(* Logix 5000 AddOnInstructionDefinition export Banner_Q90R2KU_Param_v4; software revision 33.00; part 3 of 3 *)
(* tags used below, declared in another part *)
   Q90RKU : Banner_Q90R2KU_v4;
   Port_Data : Banner_IOL_Port_v4;
   Port : DINT;
   Local_Control : DINT;
   Command_Being_Processed : BOOL;
   Update_Archive : BOOL;
   Index_Write_Inprocess : DINT;
   Inprocess_Index : DINT;
(* Banner_Q90R2KU_Param_v4, continued *)

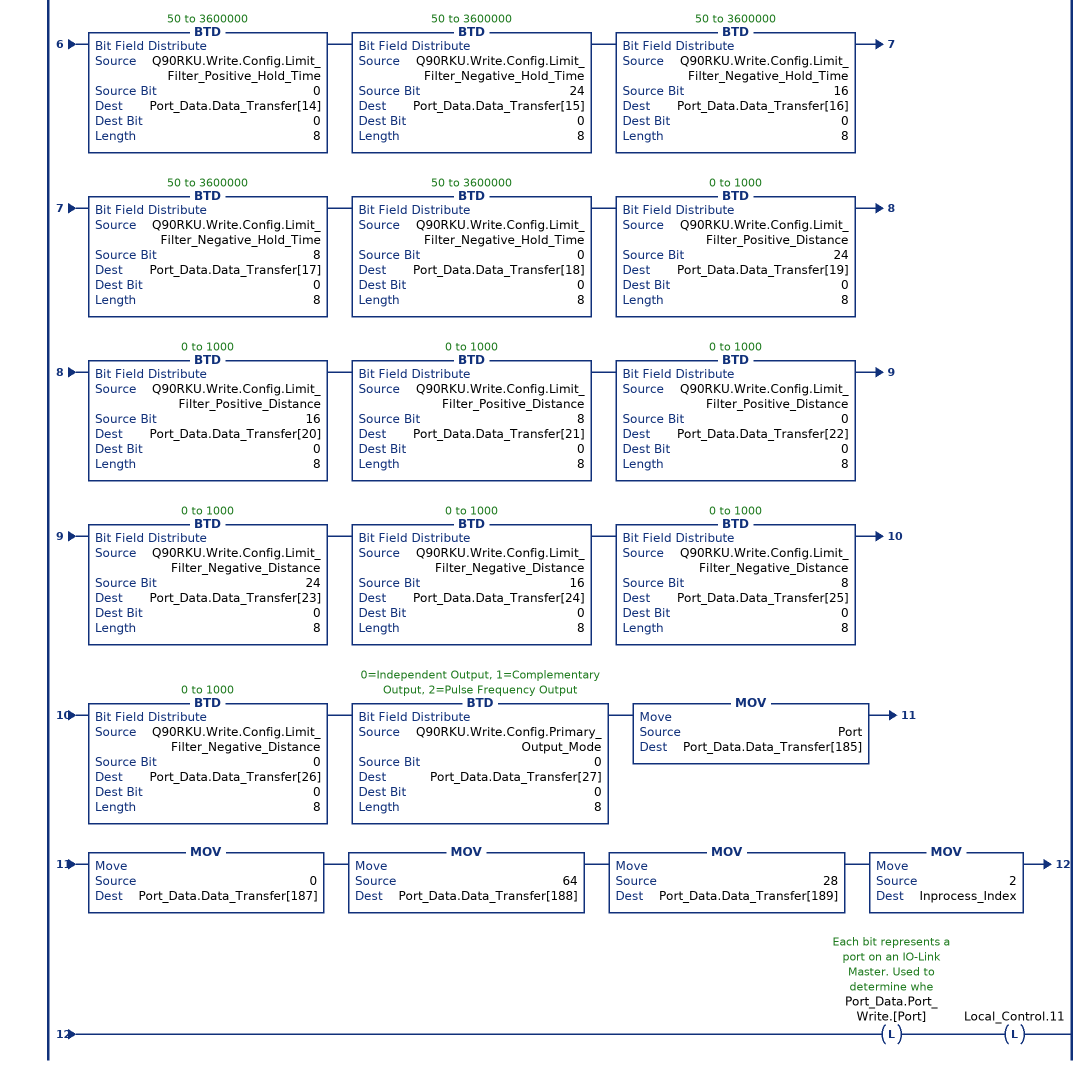
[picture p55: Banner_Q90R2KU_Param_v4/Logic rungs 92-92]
   // ************************************************************************************************************
   // Section of AOI that controls writing of the Configuration parameter (index 64).
   // ************************************************************************************************************
   92: XIC(Q90RKU.Initial_Global_Read)XIO(Command_Being_Processed)XIO(Local_Control.11)EQU(Q90RKU.Command,44)OTL(Command_Being_Processed)MOV(0,Port_Data.Data_Transfer[0])MOV(0,Port_Data.Data_Transfer[1])BTD(Q90RKU.Write.Config.Response_Speed,0,Port_Data.Data_Transfer[0],0,8)BTD(Q90RKU.Write.Config.Detection_Sensitivity,0,Port_Data.Data_Transfer[1],0,8)BTD(Q90RKU.Write.Config.LEDs_Disabled,0,Port_Data.Data_Transfer[2],0,8)BTD(Q90RKU.Write.Config.Output_Polarity,0,Port_Data.Data_Transfer[3],0,8)BTD(Q90RKU.Write.Config.PD_Measurement,0,Port_Data.Data_Transfer[4],0,8)BTD(Q90RKU.Write.Config.Remote_Input_Mode,0,Port_Data.Data_Transfer[5],0,8)BTD(Q90RKU.Write.Config.Amplitude_Threshold,24,Port_Data.Data_Transfer[6],0,8)BTD(Q90RKU.Write.Config.Amplitude_Threshold,16,Port_Data.Data_Transfer[7],0,8)BTD(Q90RKU.Write.Config.Amplitude_Threshold,8,Port_Data.Data_Transfer[8],0,8)BTD(Q90RKU.Write.Config.Amplitude_Threshold,0,Port_Data.Data_Transfer[9],0,8)BTD(Q90RKU.Write.Config.Limit_Filter_Enabled,0,Port_Data.Data_Transfer[10],0,8)BTD(Q90RKU.Write.Config.Limit_Filter_Positive_Hold_Time,24,Port_Data.Data_Transfer[11],0,8)BTD(Q90RKU.Write.Config.Limit_Filter_Positive_Hold_Time,16,Port_Data.Data_Transfer[12],0,8)BTD(Q90RKU.Write.Config.Limit_Filter_Positive_Hold_Time,8,Port_Data.Data_Transfer[13],0,8)BTD(Q90RKU.Write.Config.Limit_Filter_Positive_Hold_Time,0,Port_Data.Data_Transfer[14],0,8)BTD(Q90RKU.Write.Config.Limit_Filter_Negative_Hold_Time,24,Port_Data.Data_Transfer[15],0,8)BTD(Q90RKU.Write.Config.Limit_Filter_Negative_Hold_Time,16,Port_Data.Data_Transfer[16],0,8)BTD(Q90RKU.Write.Config.Limit_Filter_Negative_Hold_Time,8,Port_Data.Data_Transfer[17],0,8)BTD(Q90RKU.Write.Config.Limit_Filter_Negative_Hold_Time,0,Port_Data.Data_Transfer[18],0,8)BTD(Q90RKU.Write.Config.Limit_Filter_Positive_Distance,24,Port_Data.Data_Transfer[19],0,8)BTD(Q90RKU.Write.Config.Limit_Filter_Positive_Distance,16,Port_Data.Data_Transfer[20],0,8)BTD(Q90RKU.Write.Config.Limit_Filter_Positive_Distance,8,Port_Data.Data_Transfer[21],0,8)BTD(Q90RKU.Write.Config.Limit_Filter_Positive_Distance,0,Port_Data.Data_Transfer[22],0,8)BTD(Q90RKU.Write.Config.Limit_Filter_Negative_Distance,24,Port_Data.Data_Transfer[23],0,8)BTD(Q90RKU.Write.Config.Limit_Filter_Negative_Distance,16,Port_Data.Data_Transfer[24],0,8)BTD(Q90RKU.Write.Config.Limit_Filter_Negative_Distance,8,Port_Data.Data_Transfer[25],0,8)BTD(Q90RKU.Write.Config.Limit_Filter_Negative_Distance,0,Port_Data.Data_Transfer[26],0,8)BTD(Q90RKU.Write.Config.Primary_Output_Mode,0,Port_Data.Data_Transfer[27],0,8)MOV(Port,Port_Data.Data_Transfer[185])MOV(0,Port_Data.Data_Transfer[187])MOV(64,Port_Data.Data_Transfer[188])MOV(28,Port_Data.Data_Transfer[189])MOV(2,Inprocess_Index)OTL(Port_Data.Port_Write.[Port])OTL(Local_Control.11);
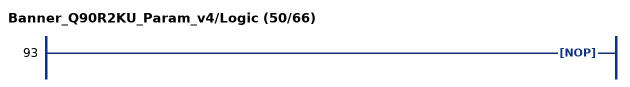
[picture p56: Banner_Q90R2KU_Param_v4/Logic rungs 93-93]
   93: NOP();
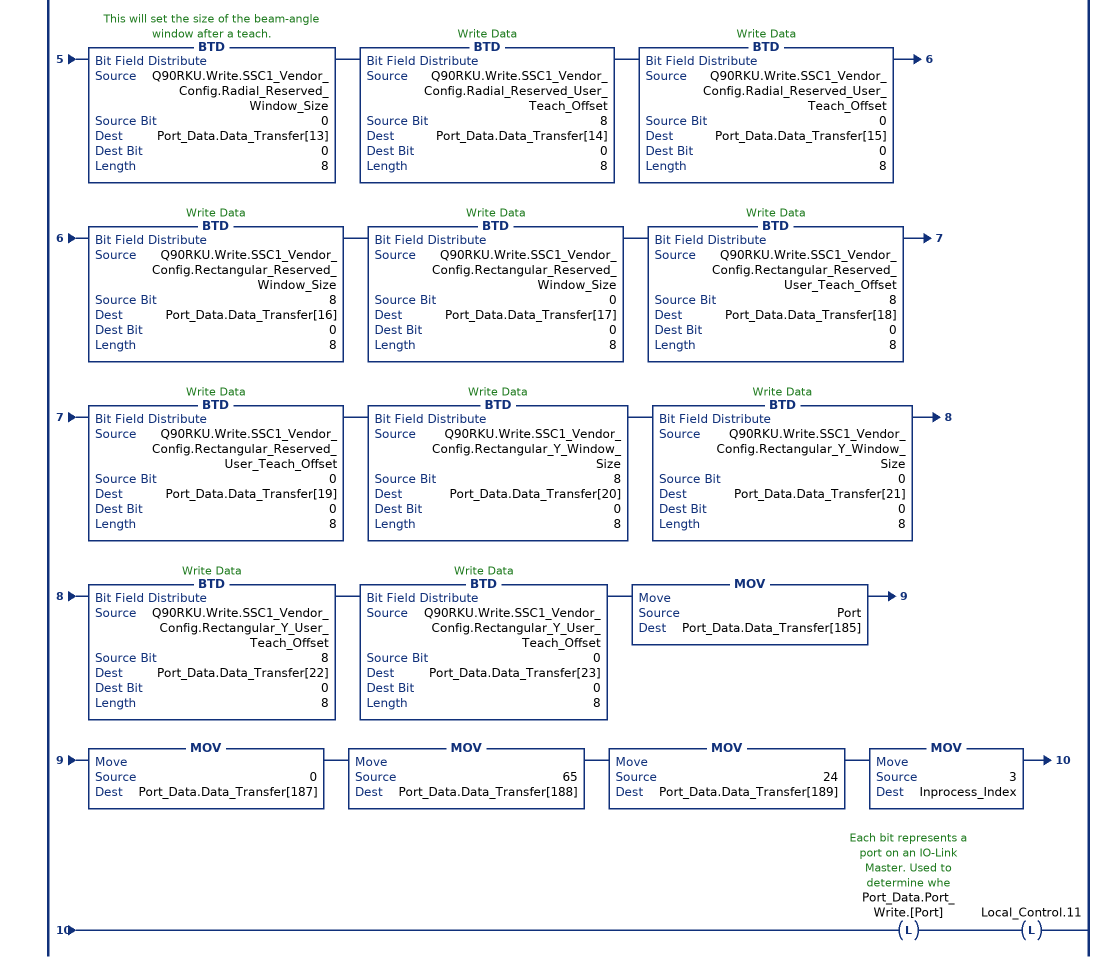
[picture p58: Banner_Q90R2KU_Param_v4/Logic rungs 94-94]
   // ************************************************************************************************************
   // Section of AOI that controls writing of the SSC1 Vendor Specific Configuration parameter (index 65).
   // ************************************************************************************************************
   94: XIC(Q90RKU.Initial_Global_Read)XIO(Command_Being_Processed)XIO(Local_Control.11)EQU(Q90RKU.Command,45)OTL(Command_Being_Processed)BTD(Q90RKU.Write.SSC1_Vendor_Config.Delay_On,24,Port_Data.Data_Transfer[0],0,8)BTD(Q90RKU.Write.SSC1_Vendor_Config.Delay_On,16,Port_Data.Data_Transfer[1],0,8)BTD(Q90RKU.Write.SSC1_Vendor_Config.Delay_On,8,Port_Data.Data_Transfer[2],0,8)BTD(Q90RKU.Write.SSC1_Vendor_Config.Delay_On,0,Port_Data.Data_Transfer[3],0,8)BTD(Q90RKU.Write.SSC1_Vendor_Config.Delay_Off,24,Port_Data.Data_Transfer[4],0,8)BTD(Q90RKU.Write.SSC1_Vendor_Config.Delay_Off,16,Port_Data.Data_Transfer[5],0,8)BTD(Q90RKU.Write.SSC1_Vendor_Config.Delay_Off,8,Port_Data.Data_Transfer[6],0,8)BTD(Q90RKU.Write.SSC1_Vendor_Config.Delay_Off,0,Port_Data.Data_Transfer[7],0,8)BTD(Q90RKU.Write.SSC1_Vendor_Config.Radial_Distance_Window_Size,8,Port_Data.Data_Transfer[8],0,8)BTD(Q90RKU.Write.SSC1_Vendor_Config.Radial_Distance_Window_Size,0,Port_Data.Data_Transfer[9],0,8)BTD(Q90RKU.Write.SSC1_Vendor_Config.Radial_Distance_User_Teach_Offset,8,Port_Data.Data_Transfer[10],0,8)BTD(Q90RKU.Write.SSC1_Vendor_Config.Radial_Distance_User_Teach_Offset,0,Port_Data.Data_Transfer[11],0,8)BTD(Q90RKU.Write.SSC1_Vendor_Config.Radial_Reserved_Window_Size,8,Port_Data.Data_Transfer[12],0,8)BTD(Q90RKU.Write.SSC1_Vendor_Config.Radial_Reserved_Window_Size,0,Port_Data.Data_Transfer[13],0,8)BTD(Q90RKU.Write.SSC1_Vendor_Config.Radial_Reserved_User_Teach_Offset,8,Port_Data.Data_Transfer[14],0,8)BTD(Q90RKU.Write.SSC1_Vendor_Config.Radial_Reserved_User_Teach_Offset,0,Port_Data.Data_Transfer[15],0,8)BTD(Q90RKU.Write.SSC1_Vendor_Config.Rectangular_Reserved_Window_Size,8,Port_Data.Data_Transfer[16],0,8)BTD(Q90RKU.Write.SSC1_Vendor_Config.Rectangular_Reserved_Window_Size,0,Port_Data.Data_Transfer[17],0,8)BTD(Q90RKU.Write.SSC1_Vendor_Config.Rectangular_Reserved_User_Teach_Offset,8,Port_Data.Data_Transfer[18],0,8)BTD(Q90RKU.Write.SSC1_Vendor_Config.Rectangular_Reserved_User_Teach_Offset,0,Port_Data.Data_Transfer[19],0,8)BTD(Q90RKU.Write.SSC1_Vendor_Config.Rectangular_Y_Window_Size,8,Port_Data.Data_Transfer[20],0,8)BTD(Q90RKU.Write.SSC1_Vendor_Config.Rectangular_Y_Window_Size,0,Port_Data.Data_Transfer[21],0,8)BTD(Q90RKU.Write.SSC1_Vendor_Config.Rectangular_Y_User_Teach_Offset,8,Port_Data.Data_Transfer[22],0,8)BTD(Q90RKU.Write.SSC1_Vendor_Config.Rectangular_Y_User_Teach_Offset,0,Port_Data.Data_Transfer[23],0,8)MOV(Port,Port_Data.Data_Transfer[185])MOV(0,Port_Data.Data_Transfer[187])MOV(65,Port_Data.Data_Transfer[188])MOV(24,Port_Data.Data_Transfer[189])MOV(3,Inprocess_Index)OTL(Port_Data.Port_Write.[Port])OTL(Local_Control.11);
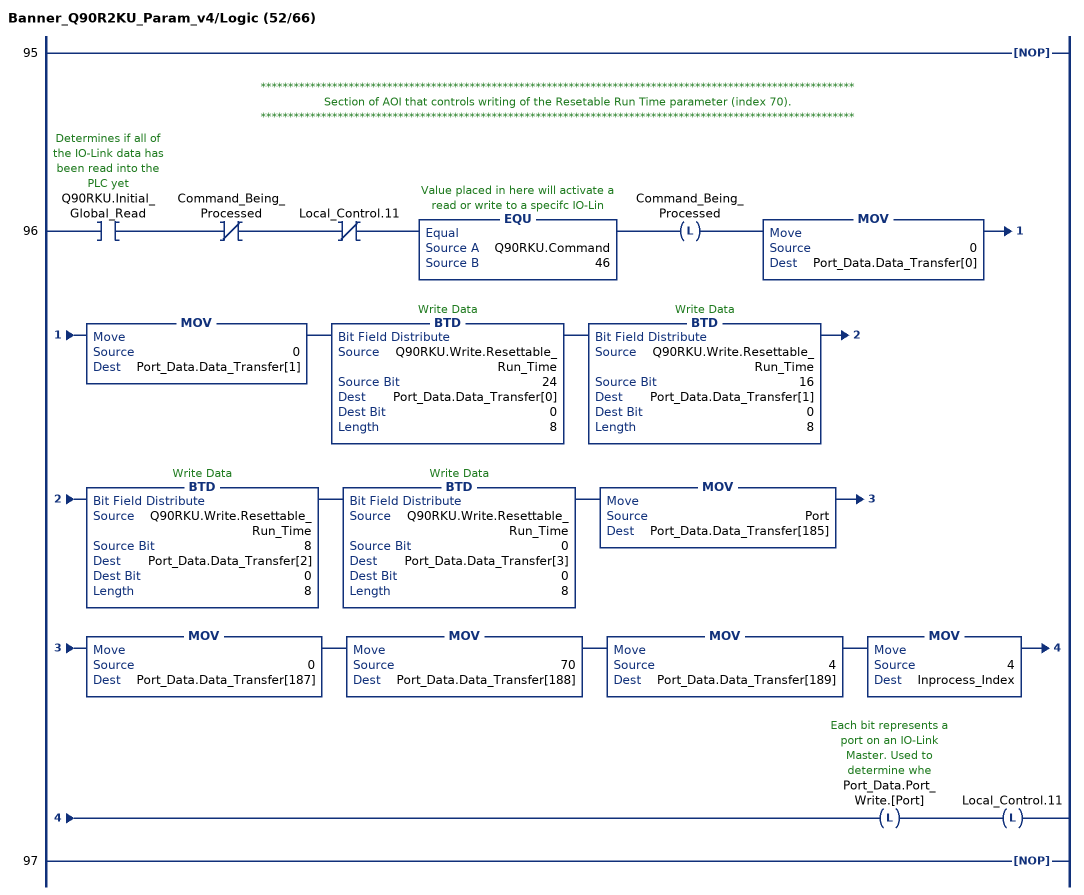
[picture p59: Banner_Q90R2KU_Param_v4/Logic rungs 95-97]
   95: NOP();
   // ************************************************************************************************************
   // Section of AOI that controls writing of the Resetable Run Time parameter (index 70).
   // ************************************************************************************************************
   96: XIC(Q90RKU.Initial_Global_Read)XIO(Command_Being_Processed)XIO(Local_Control.11)EQU(Q90RKU.Command,46)OTL(Command_Being_Processed)MOV(0,Port_Data.Data_Transfer[0])MOV(0,Port_Data.Data_Transfer[1])BTD(Q90RKU.Write.Resettable_Run_Time,24,Port_Data.Data_Transfer[0],0,8)BTD(Q90RKU.Write.Resettable_Run_Time,16,Port_Data.Data_Transfer[1],0,8)BTD(Q90RKU.Write.Resettable_Run_Time,8,Port_Data.Data_Transfer[2],0,8)BTD(Q90RKU.Write.Resettable_Run_Time,0,Port_Data.Data_Transfer[3],0,8)MOV(Port,Port_Data.Data_Transfer[185])MOV(0,Port_Data.Data_Transfer[187])MOV(70,Port_Data.Data_Transfer[188])MOV(4,Port_Data.Data_Transfer[189])MOV(4,Inprocess_Index)OTL(Port_Data.Port_Write.[Port])OTL(Local_Control.11);
   97: NOP();
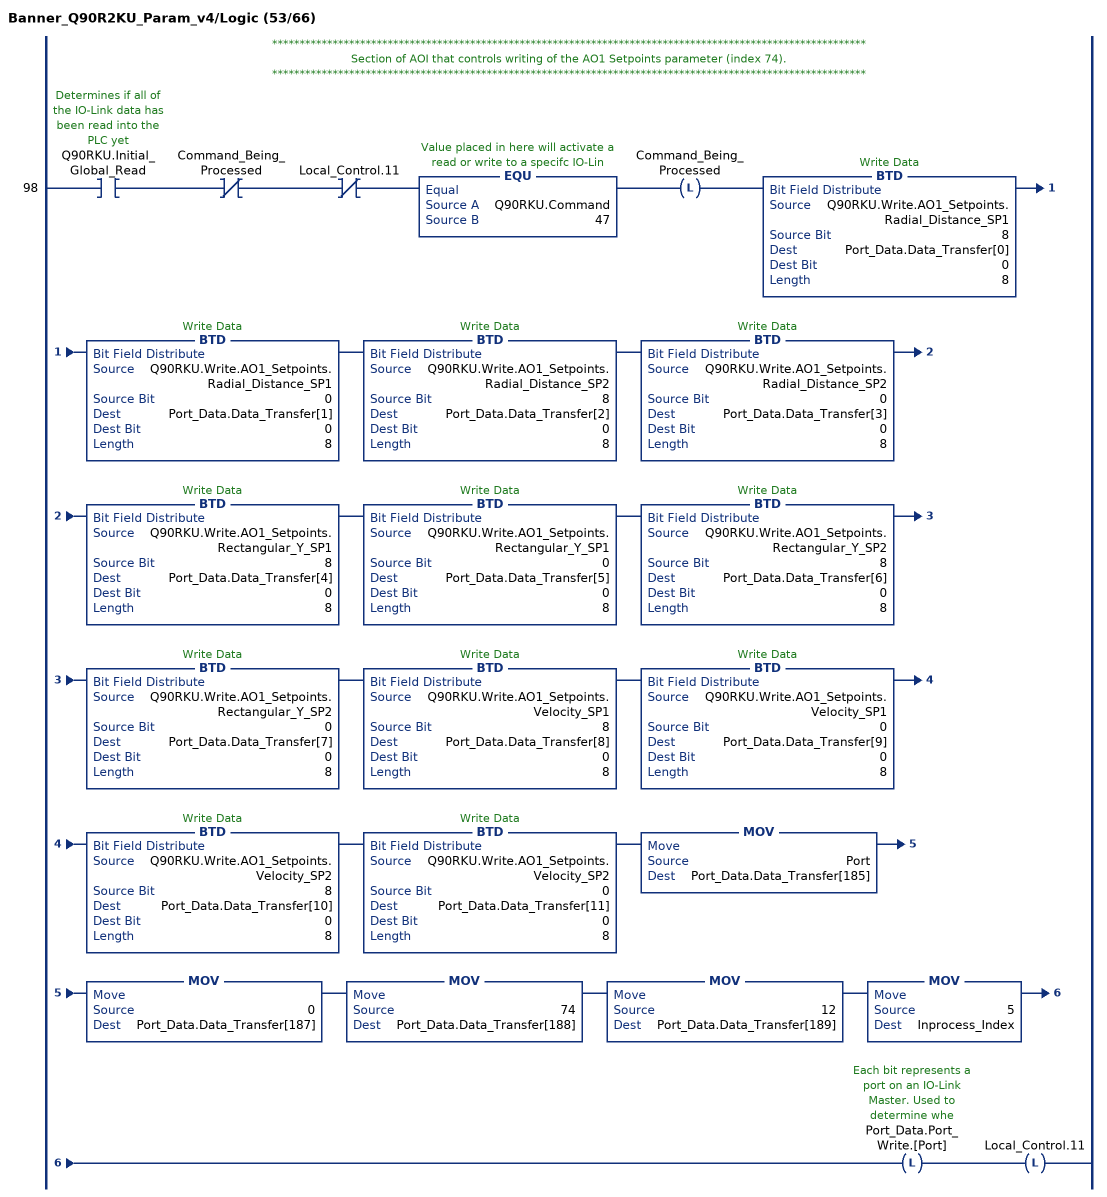
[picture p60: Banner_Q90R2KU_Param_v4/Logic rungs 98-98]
   // ************************************************************************************************************
   // Section of AOI that controls writing of the AO1 Setpoints parameter (index 74).
   // ************************************************************************************************************
   98: XIC(Q90RKU.Initial_Global_Read)XIO(Command_Being_Processed)XIO(Local_Control.11)EQU(Q90RKU.Command,47)OTL(Command_Being_Processed)BTD(Q90RKU.Write.AO1_Setpoints.Radial_Distance_SP1,8,Port_Data.Data_Transfer[0],0,8)BTD(Q90RKU.Write.AO1_Setpoints.Radial_Distance_SP1,0,Port_Data.Data_Transfer[1],0,8)BTD(Q90RKU.Write.AO1_Setpoints.Radial_Distance_SP2,8,Port_Data.Data_Transfer[2],0,8)BTD(Q90RKU.Write.AO1_Setpoints.Radial_Distance_SP2,0,Port_Data.Data_Transfer[3],0,8)BTD(Q90RKU.Write.AO1_Setpoints.Rectangular_Y_SP1,8,Port_Data.Data_Transfer[4],0,8)BTD(Q90RKU.Write.AO1_Setpoints.Rectangular_Y_SP1,0,Port_Data.Data_Transfer[5],0,8)BTD(Q90RKU.Write.AO1_Setpoints.Rectangular_Y_SP2,8,Port_Data.Data_Transfer[6],0,8)BTD(Q90RKU.Write.AO1_Setpoints.Rectangular_Y_SP2,0,Port_Data.Data_Transfer[7],0,8)BTD(Q90RKU.Write.AO1_Setpoints.Velocity_SP1,8,Port_Data.Data_Transfer[8],0,8)BTD(Q90RKU.Write.AO1_Setpoints.Velocity_SP1,0,Port_Data.Data_Transfer[9],0,8)BTD(Q90RKU.Write.AO1_Setpoints.Velocity_SP2,8,Port_Data.Data_Transfer[10],0,8)BTD(Q90RKU.Write.AO1_Setpoints.Velocity_SP2,0,Port_Data.Data_Transfer[11],0,8)MOV(Port,Port_Data.Data_Transfer[185])MOV(0,Port_Data.Data_Transfer[187])MOV(74,Port_Data.Data_Transfer[188])MOV(12,Port_Data.Data_Transfer[189])MOV(5,Inprocess_Index)OTL(Port_Data.Port_Write.[Port])OTL(Local_Control.11);
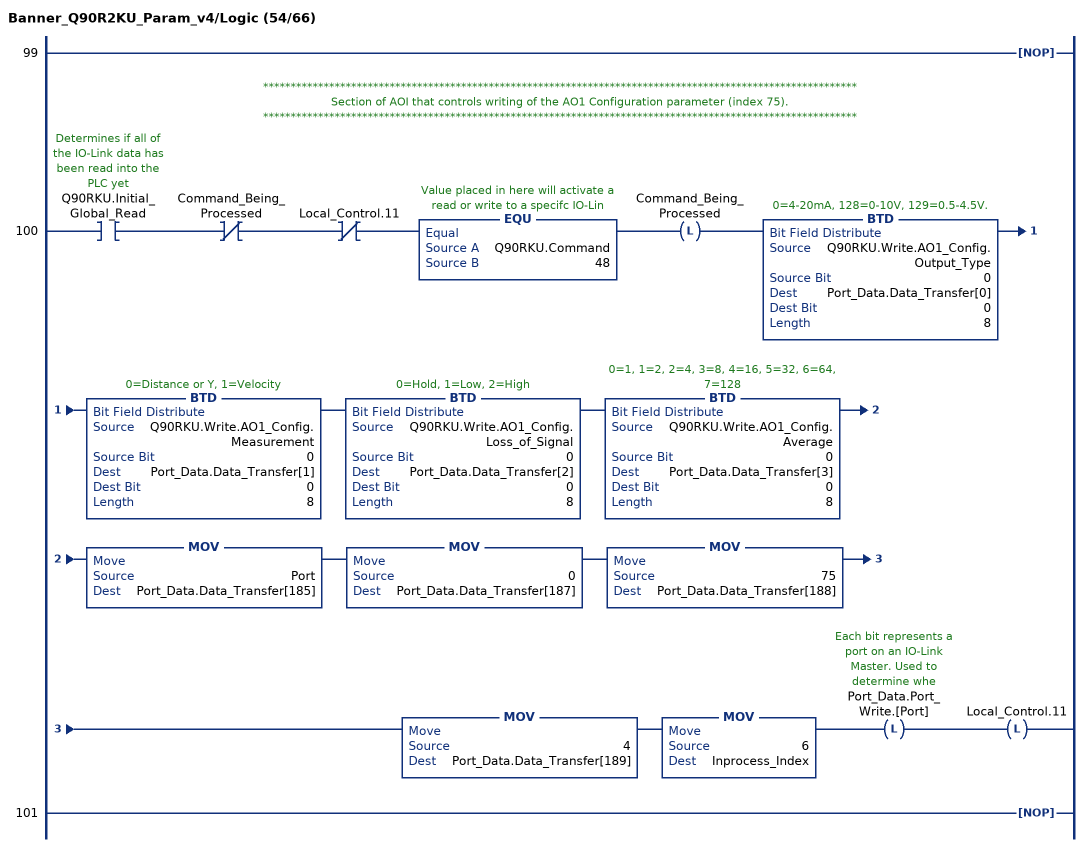
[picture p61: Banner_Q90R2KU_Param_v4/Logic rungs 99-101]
   99: NOP();
   // ************************************************************************************************************
   // Section of AOI that controls writing of the AO1 Configuration parameter (index 75).
   // ************************************************************************************************************
   100: XIC(Q90RKU.Initial_Global_Read)XIO(Command_Being_Processed)XIO(Local_Control.11)EQU(Q90RKU.Command,48)OTL(Command_Being_Processed)BTD(Q90RKU.Write.AO1_Config.Output_Type,0,Port_Data.Data_Transfer[0],0,8)BTD(Q90RKU.Write.AO1_Config.Measurement,0,Port_Data.Data_Transfer[1],0,8)BTD(Q90RKU.Write.AO1_Config.Loss_of_Signal,0,Port_Data.Data_Transfer[2],0,8)BTD(Q90RKU.Write.AO1_Config.Average,0,Port_Data.Data_Transfer[3],0,8)MOV(Port,Port_Data.Data_Transfer[185])MOV(0,Port_Data.Data_Transfer[187])MOV(75,Port_Data.Data_Transfer[188])MOV(4,Port_Data.Data_Transfer[189])MOV(6,Inprocess_Index)OTL(Port_Data.Port_Write.[Port])OTL(Local_Control.11);
   101: NOP();
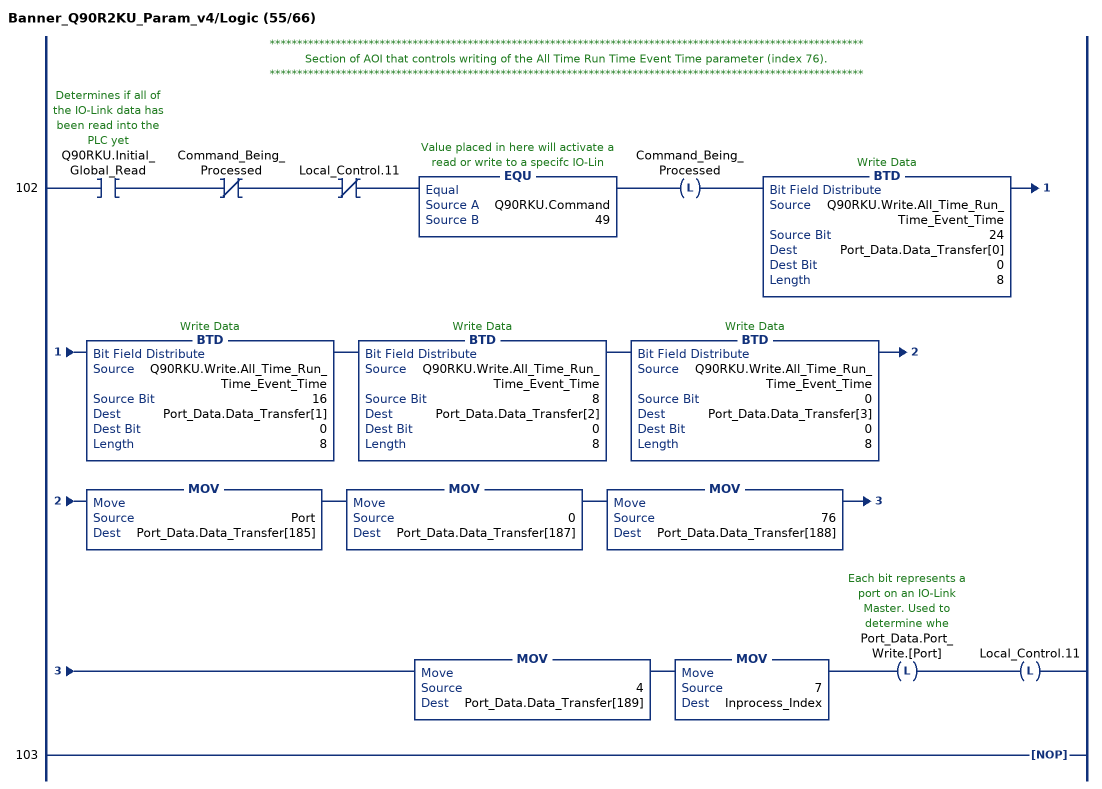
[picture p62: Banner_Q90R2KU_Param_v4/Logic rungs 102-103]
   // ************************************************************************************************************
   // Section of AOI that controls writing of the All Time Run Time Event Time parameter (index 76).
   // ************************************************************************************************************
   102: XIC(Q90RKU.Initial_Global_Read)XIO(Command_Being_Processed)XIO(Local_Control.11)EQU(Q90RKU.Command,49)OTL(Command_Being_Processed)BTD(Q90RKU.Write.All_Time_Run_Time_Event_Time,24,Port_Data.Data_Transfer[0],0,8)BTD(Q90RKU.Write.All_Time_Run_Time_Event_Time,16,Port_Data.Data_Transfer[1],0,8)BTD(Q90RKU.Write.All_Time_Run_Time_Event_Time,8,Port_Data.Data_Transfer[2],0,8)BTD(Q90RKU.Write.All_Time_Run_Time_Event_Time,0,Port_Data.Data_Transfer[3],0,8)MOV(Port,Port_Data.Data_Transfer[185])MOV(0,Port_Data.Data_Transfer[187])MOV(76,Port_Data.Data_Transfer[188])MOV(4,Port_Data.Data_Transfer[189])MOV(7,Inprocess_Index)OTL(Port_Data.Port_Write.[Port])OTL(Local_Control.11);
   103: NOP();
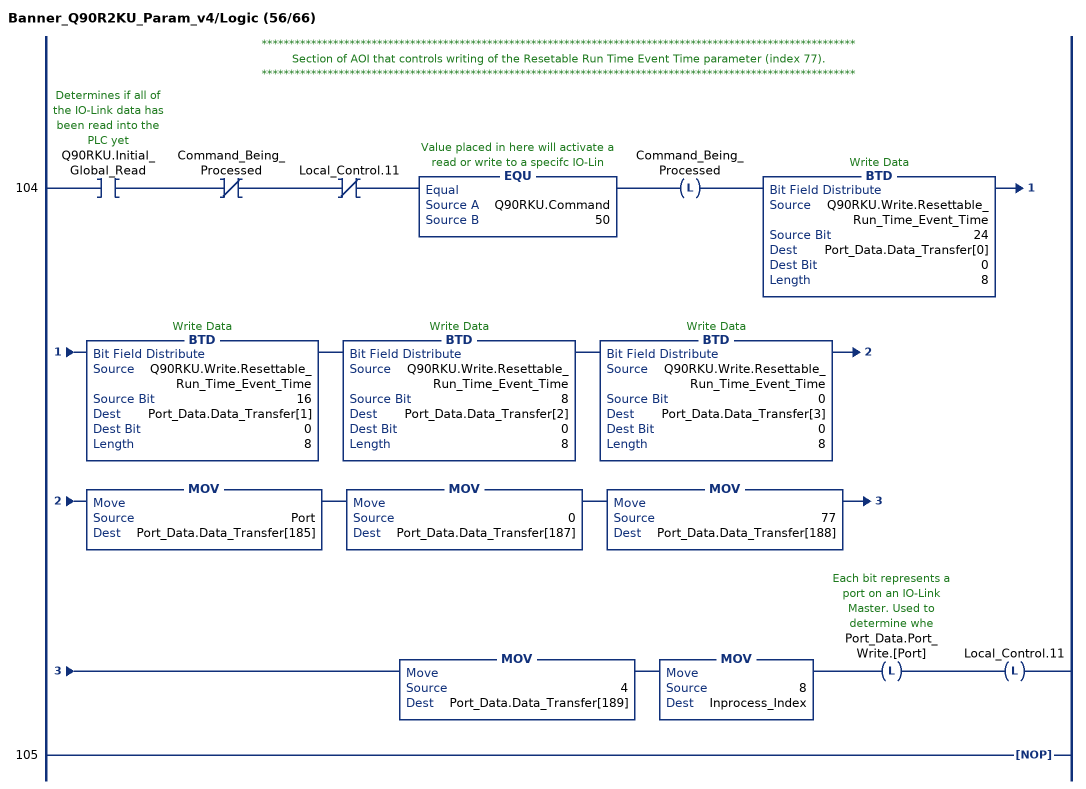
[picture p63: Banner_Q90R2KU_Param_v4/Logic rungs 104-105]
   // ************************************************************************************************************
   // Section of AOI that controls writing of the Resetable Run Time Event Time parameter (index 77).
   // ************************************************************************************************************
   104: XIC(Q90RKU.Initial_Global_Read)XIO(Command_Being_Processed)XIO(Local_Control.11)EQU(Q90RKU.Command,50)OTL(Command_Being_Processed)BTD(Q90RKU.Write.Resettable_Run_Time_Event_Time,24,Port_Data.Data_Transfer[0],0,8)BTD(Q90RKU.Write.Resettable_Run_Time_Event_Time,16,Port_Data.Data_Transfer[1],0,8)BTD(Q90RKU.Write.Resettable_Run_Time_Event_Time,8,Port_Data.Data_Transfer[2],0,8)BTD(Q90RKU.Write.Resettable_Run_Time_Event_Time,0,Port_Data.Data_Transfer[3],0,8)MOV(Port,Port_Data.Data_Transfer[185])MOV(0,Port_Data.Data_Transfer[187])MOV(77,Port_Data.Data_Transfer[188])MOV(4,Port_Data.Data_Transfer[189])MOV(8,Inprocess_Index)OTL(Port_Data.Port_Write.[Port])OTL(Local_Control.11);
   105: NOP();
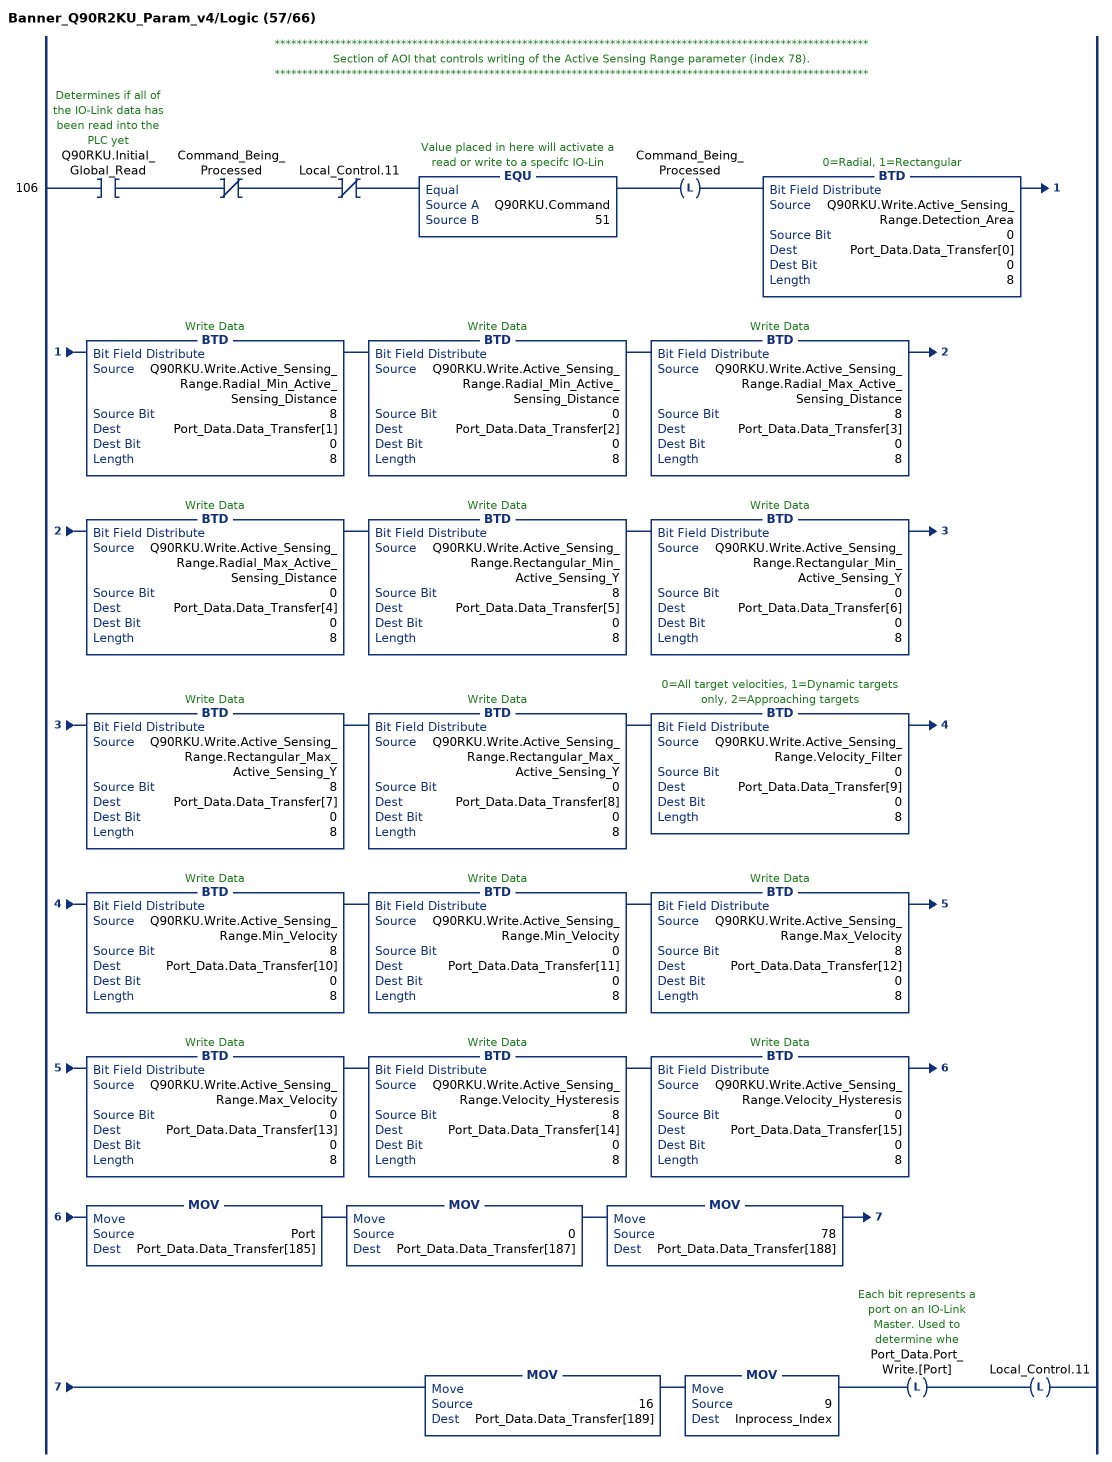
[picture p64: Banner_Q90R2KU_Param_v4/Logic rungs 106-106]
   // ************************************************************************************************************
   // Section of AOI that controls writing of the Active Sensing Range parameter (index 78).
   // ************************************************************************************************************
   106: XIC(Q90RKU.Initial_Global_Read)XIO(Command_Being_Processed)XIO(Local_Control.11)EQU(Q90RKU.Command,51)OTL(Command_Being_Processed)BTD(Q90RKU.Write.Active_Sensing_Range.Detection_Area,0,Port_Data.Data_Transfer[0],0,8)BTD(Q90RKU.Write.Active_Sensing_Range.Radial_Min_Active_Sensing_Distance,8,Port_Data.Data_Transfer[1],0,8)BTD(Q90RKU.Write.Active_Sensing_Range.Radial_Min_Active_Sensing_Distance,0,Port_Data.Data_Transfer[2],0,8)BTD(Q90RKU.Write.Active_Sensing_Range.Radial_Max_Active_Sensing_Distance,8,Port_Data.Data_Transfer[3],0,8)BTD(Q90RKU.Write.Active_Sensing_Range.Radial_Max_Active_Sensing_Distance,0,Port_Data.Data_Transfer[4],0,8)BTD(Q90RKU.Write.Active_Sensing_Range.Rectangular_Min_Active_Sensing_Y,8,Port_Data.Data_Transfer[5],0,8)BTD(Q90RKU.Write.Active_Sensing_Range.Rectangular_Min_Active_Sensing_Y,0,Port_Data.Data_Transfer[6],0,8)BTD(Q90RKU.Write.Active_Sensing_Range.Rectangular_Max_Active_Sensing_Y,8,Port_Data.Data_Transfer[7],0,8)BTD(Q90RKU.Write.Active_Sensing_Range.Rectangular_Max_Active_Sensing_Y,0,Port_Data.Data_Transfer[8],0,8)BTD(Q90RKU.Write.Active_Sensing_Range.Velocity_Filter,0,Port_Data.Data_Transfer[9],0,8)BTD(Q90RKU.Write.Active_Sensing_Range.Min_Velocity,8,Port_Data.Data_Transfer[10],0,8)BTD(Q90RKU.Write.Active_Sensing_Range.Min_Velocity,0,Port_Data.Data_Transfer[11],0,8)BTD(Q90RKU.Write.Active_Sensing_Range.Max_Velocity,8,Port_Data.Data_Transfer[12],0,8)BTD(Q90RKU.Write.Active_Sensing_Range.Max_Velocity,0,Port_Data.Data_Transfer[13],0,8)BTD(Q90RKU.Write.Active_Sensing_Range.Velocity_Hysteresis,8,Port_Data.Data_Transfer[14],0,8)BTD(Q90RKU.Write.Active_Sensing_Range.Velocity_Hysteresis,0,Port_Data.Data_Transfer[15],0,8)MOV(Port,Port_Data.Data_Transfer[185])MOV(0,Port_Data.Data_Transfer[187])MOV(78,Port_Data.Data_Transfer[188])MOV(16,Port_Data.Data_Transfer[189])MOV(9,Inprocess_Index)OTL(Port_Data.Port_Write.[Port])OTL(Local_Control.11);
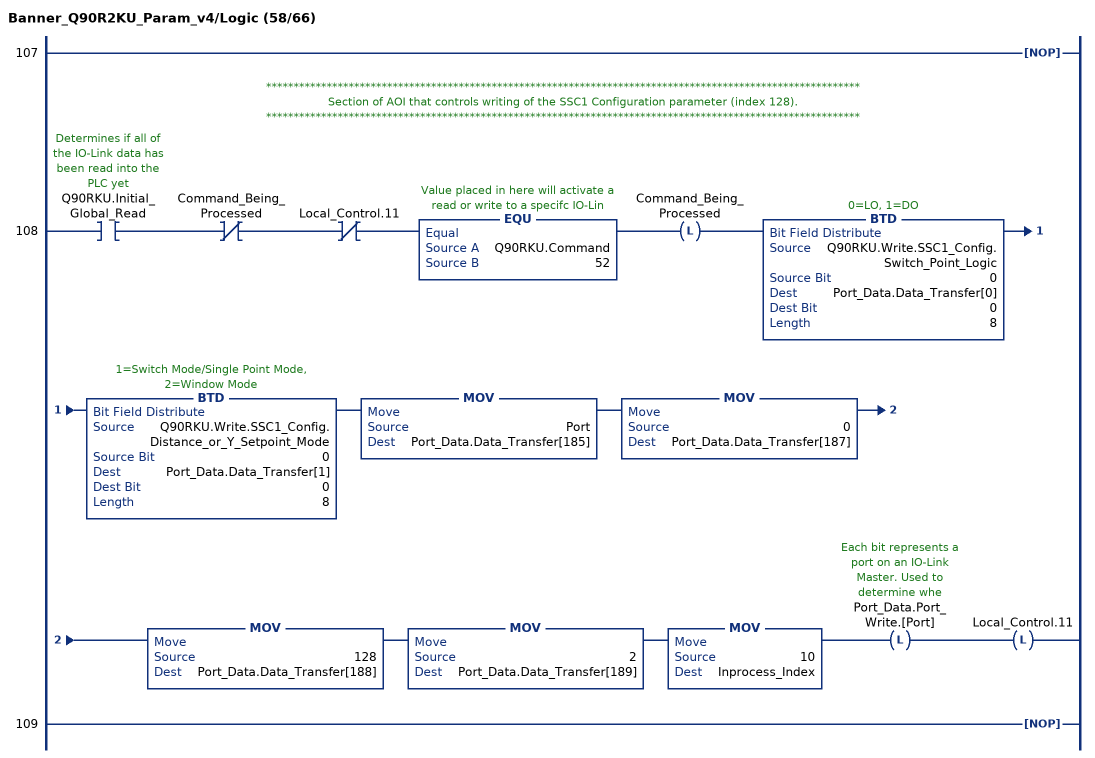
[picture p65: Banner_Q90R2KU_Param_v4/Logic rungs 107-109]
   107: NOP();
   // ************************************************************************************************************
   // Section of AOI that controls writing of the SSC1 Configuration parameter (index 128).
   // ************************************************************************************************************
   108: XIC(Q90RKU.Initial_Global_Read)XIO(Command_Being_Processed)XIO(Local_Control.11)EQU(Q90RKU.Command,52)OTL(Command_Being_Processed)BTD(Q90RKU.Write.SSC1_Config.Switch_Point_Logic,0,Port_Data.Data_Transfer[0],0,8)BTD(Q90RKU.Write.SSC1_Config.Distance_or_Y_Setpoint_Mode,0,Port_Data.Data_Transfer[1],0,8)MOV(Port,Port_Data.Data_Transfer[185])MOV(0,Port_Data.Data_Transfer[187])MOV(128,Port_Data.Data_Transfer[188])MOV(2,Port_Data.Data_Transfer[189])MOV(10,Inprocess_Index)OTL(Port_Data.Port_Write.[Port])OTL(Local_Control.11);
   109: NOP();
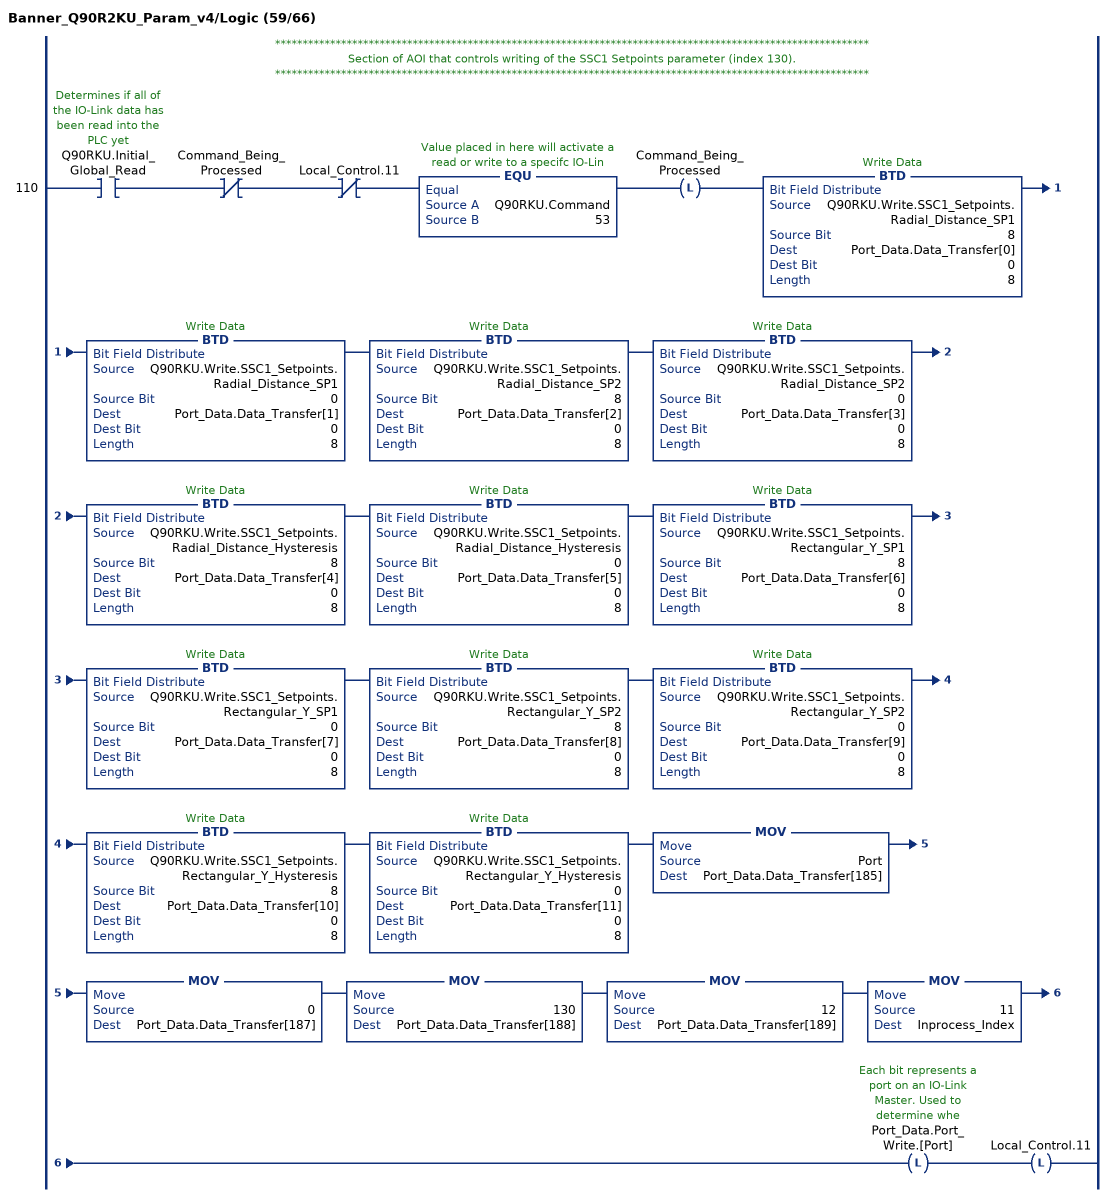
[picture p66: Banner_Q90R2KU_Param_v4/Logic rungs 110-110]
   // ************************************************************************************************************
   // Section of AOI that controls writing of the SSC1 Setpoints parameter (index 130).
   // ************************************************************************************************************
   110: XIC(Q90RKU.Initial_Global_Read)XIO(Command_Being_Processed)XIO(Local_Control.11)EQU(Q90RKU.Command,53)OTL(Command_Being_Processed)BTD(Q90RKU.Write.SSC1_Setpoints.Radial_Distance_SP1,8,Port_Data.Data_Transfer[0],0,8)BTD(Q90RKU.Write.SSC1_Setpoints.Radial_Distance_SP1,0,Port_Data.Data_Transfer[1],0,8)BTD(Q90RKU.Write.SSC1_Setpoints.Radial_Distance_SP2,8,Port_Data.Data_Transfer[2],0,8)BTD(Q90RKU.Write.SSC1_Setpoints.Radial_Distance_SP2,0,Port_Data.Data_Transfer[3],0,8)BTD(Q90RKU.Write.SSC1_Setpoints.Radial_Distance_Hysteresis,8,Port_Data.Data_Transfer[4],0,8)BTD(Q90RKU.Write.SSC1_Setpoints.Radial_Distance_Hysteresis,0,Port_Data.Data_Transfer[5],0,8)BTD(Q90RKU.Write.SSC1_Setpoints.Rectangular_Y_SP1,8,Port_Data.Data_Transfer[6],0,8)BTD(Q90RKU.Write.SSC1_Setpoints.Rectangular_Y_SP1,0,Port_Data.Data_Transfer[7],0,8)BTD(Q90RKU.Write.SSC1_Setpoints.Rectangular_Y_SP2,8,Port_Data.Data_Transfer[8],0,8)BTD(Q90RKU.Write.SSC1_Setpoints.Rectangular_Y_SP2,0,Port_Data.Data_Transfer[9],0,8)BTD(Q90RKU.Write.SSC1_Setpoints.Rectangular_Y_Hysteresis,8,Port_Data.Data_Transfer[10],0,8)BTD(Q90RKU.Write.SSC1_Setpoints.Rectangular_Y_Hysteresis,0,Port_Data.Data_Transfer[11],0,8)MOV(Port,Port_Data.Data_Transfer[185])MOV(0,Port_Data.Data_Transfer[187])MOV(130,Port_Data.Data_Transfer[188])MOV(12,Port_Data.Data_Transfer[189])MOV(11,Inprocess_Index)OTL(Port_Data.Port_Write.[Port])OTL(Local_Control.11);
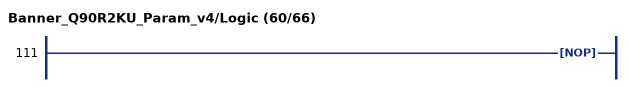
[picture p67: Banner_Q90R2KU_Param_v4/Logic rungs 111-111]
   111: NOP();
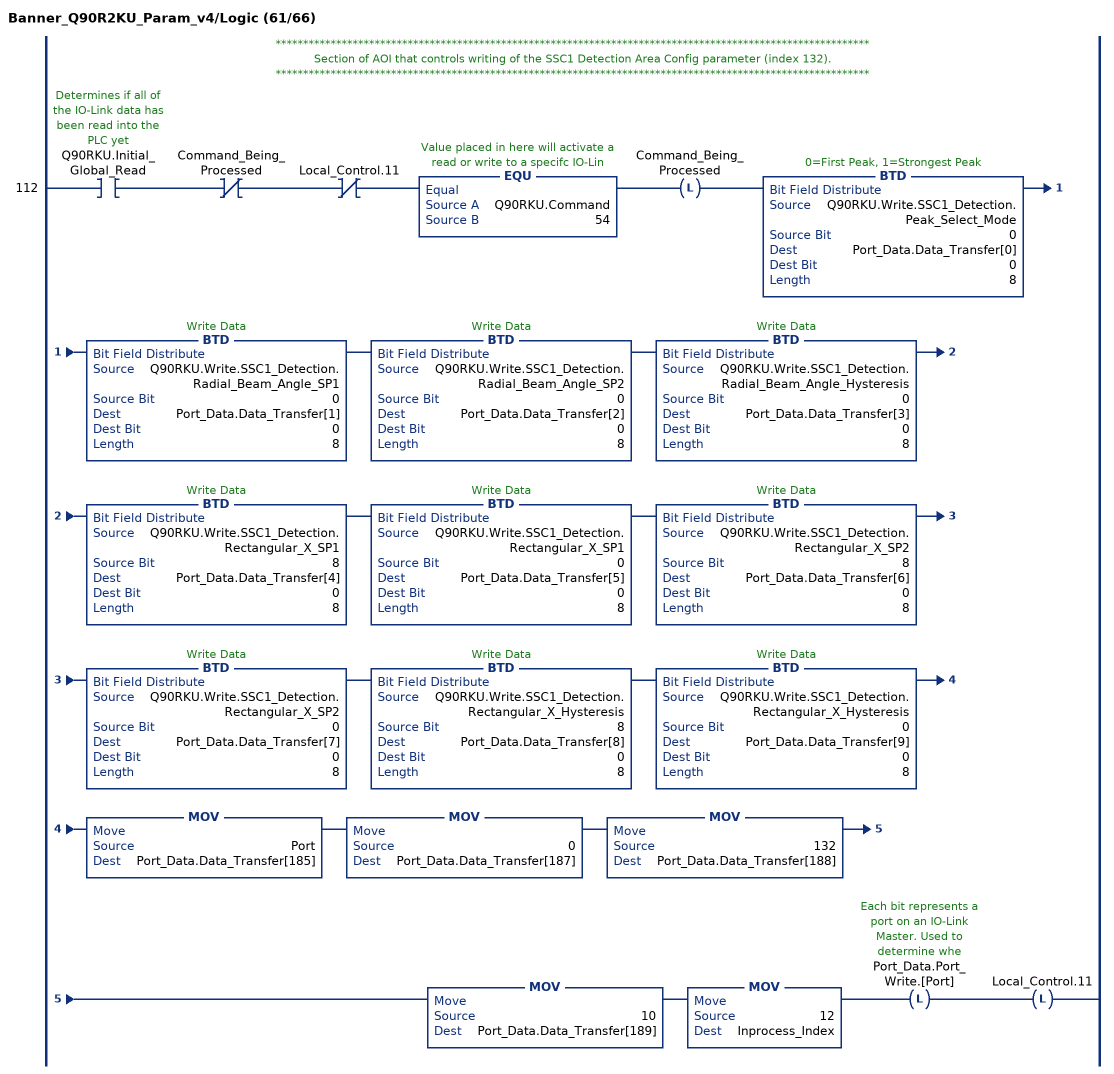
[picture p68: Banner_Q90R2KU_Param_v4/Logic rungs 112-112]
   // ************************************************************************************************************
   // Section of AOI that controls writing of the SSC1 Detection Area Config parameter (index 132).
   // ************************************************************************************************************
   112: XIC(Q90RKU.Initial_Global_Read)XIO(Command_Being_Processed)XIO(Local_Control.11)EQU(Q90RKU.Command,54)OTL(Command_Being_Processed)BTD(Q90RKU.Write.SSC1_Detection.Peak_Select_Mode,0,Port_Data.Data_Transfer[0],0,8)BTD(Q90RKU.Write.SSC1_Detection.Radial_Beam_Angle_SP1,0,Port_Data.Data_Transfer[1],0,8)BTD(Q90RKU.Write.SSC1_Detection.Radial_Beam_Angle_SP2,0,Port_Data.Data_Transfer[2],0,8)BTD(Q90RKU.Write.SSC1_Detection.Radial_Beam_Angle_Hysteresis,0,Port_Data.Data_Transfer[3],0,8)BTD(Q90RKU.Write.SSC1_Detection.Rectangular_X_SP1,8,Port_Data.Data_Transfer[4],0,8)BTD(Q90RKU.Write.SSC1_Detection.Rectangular_X_SP1,0,Port_Data.Data_Transfer[5],0,8)BTD(Q90RKU.Write.SSC1_Detection.Rectangular_X_SP2,8,Port_Data.Data_Transfer[6],0,8)BTD(Q90RKU.Write.SSC1_Detection.Rectangular_X_SP2,0,Port_Data.Data_Transfer[7],0,8)BTD(Q90RKU.Write.SSC1_Detection.Rectangular_X_Hysteresis,8,Port_Data.Data_Transfer[8],0,8)BTD(Q90RKU.Write.SSC1_Detection.Rectangular_X_Hysteresis,0,Port_Data.Data_Transfer[9],0,8)MOV(Port,Port_Data.Data_Transfer[185])MOV(0,Port_Data.Data_Transfer[187])MOV(132,Port_Data.Data_Transfer[188])MOV(10,Port_Data.Data_Transfer[189])MOV(12,Inprocess_Index)OTL(Port_Data.Port_Write.[Port])OTL(Local_Control.11);
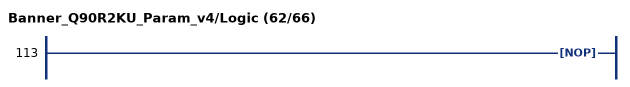
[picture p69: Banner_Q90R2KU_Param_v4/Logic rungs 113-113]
   113: NOP();
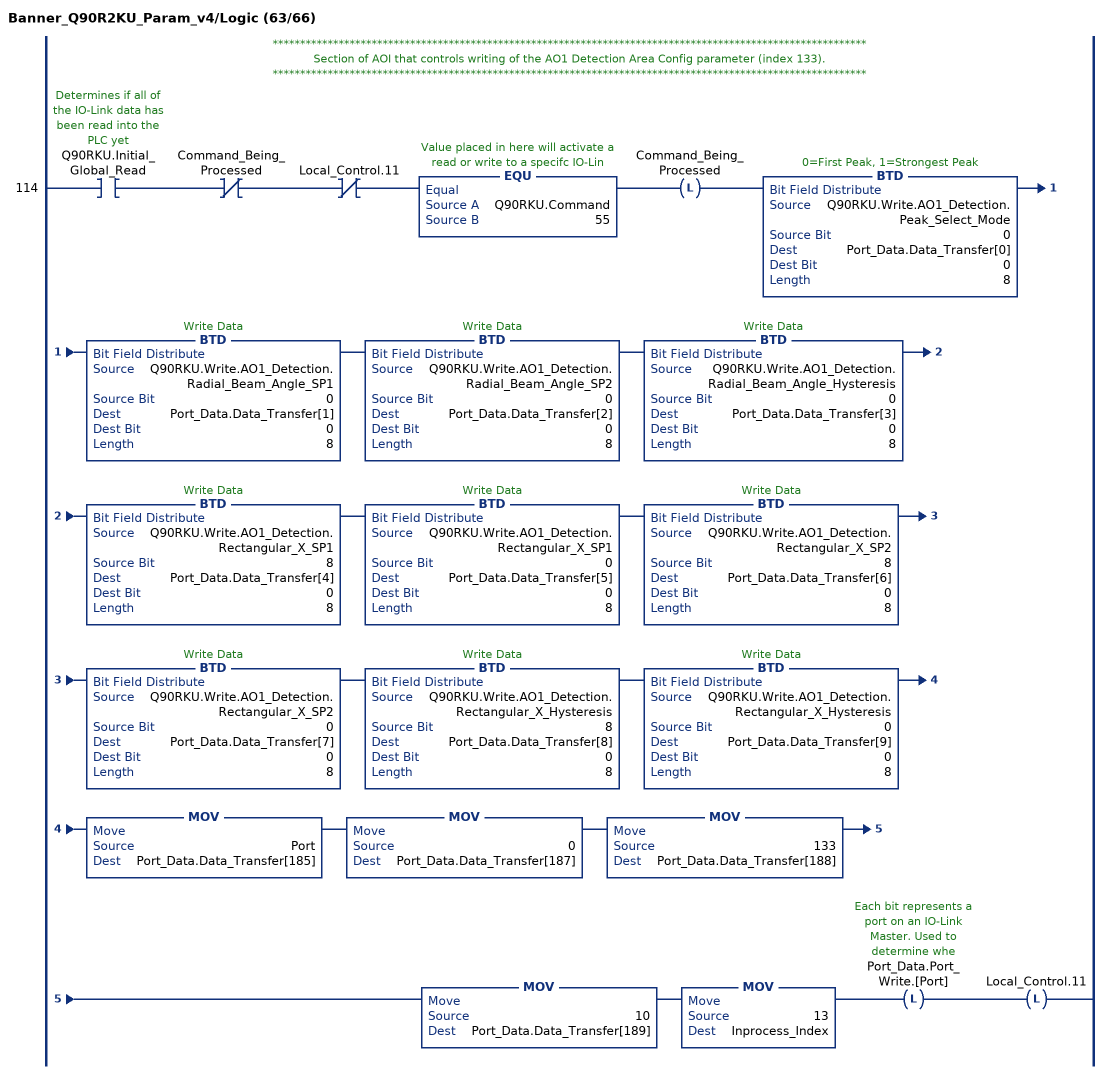
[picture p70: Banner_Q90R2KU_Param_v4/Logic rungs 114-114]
   // ************************************************************************************************************
   // Section of AOI that controls writing of the AO1 Detection Area Config parameter (index 133).
   // ************************************************************************************************************
   114: XIC(Q90RKU.Initial_Global_Read)XIO(Command_Being_Processed)XIO(Local_Control.11)EQU(Q90RKU.Command,55)OTL(Command_Being_Processed)BTD(Q90RKU.Write.AO1_Detection.Peak_Select_Mode,0,Port_Data.Data_Transfer[0],0,8)BTD(Q90RKU.Write.AO1_Detection.Radial_Beam_Angle_SP1,0,Port_Data.Data_Transfer[1],0,8)BTD(Q90RKU.Write.AO1_Detection.Radial_Beam_Angle_SP2,0,Port_Data.Data_Transfer[2],0,8)BTD(Q90RKU.Write.AO1_Detection.Radial_Beam_Angle_Hysteresis,0,Port_Data.Data_Transfer[3],0,8)BTD(Q90RKU.Write.AO1_Detection.Rectangular_X_SP1,8,Port_Data.Data_Transfer[4],0,8)BTD(Q90RKU.Write.AO1_Detection.Rectangular_X_SP1,0,Port_Data.Data_Transfer[5],0,8)BTD(Q90RKU.Write.AO1_Detection.Rectangular_X_SP2,8,Port_Data.Data_Transfer[6],0,8)BTD(Q90RKU.Write.AO1_Detection.Rectangular_X_SP2,0,Port_Data.Data_Transfer[7],0,8)BTD(Q90RKU.Write.AO1_Detection.Rectangular_X_Hysteresis,8,Port_Data.Data_Transfer[8],0,8)BTD(Q90RKU.Write.AO1_Detection.Rectangular_X_Hysteresis,0,Port_Data.Data_Transfer[9],0,8)MOV(Port,Port_Data.Data_Transfer[185])MOV(0,Port_Data.Data_Transfer[187])MOV(133,Port_Data.Data_Transfer[188])MOV(10,Port_Data.Data_Transfer[189])MOV(13,Inprocess_Index)OTL(Port_Data.Port_Write.[Port])OTL(Local_Control.11);
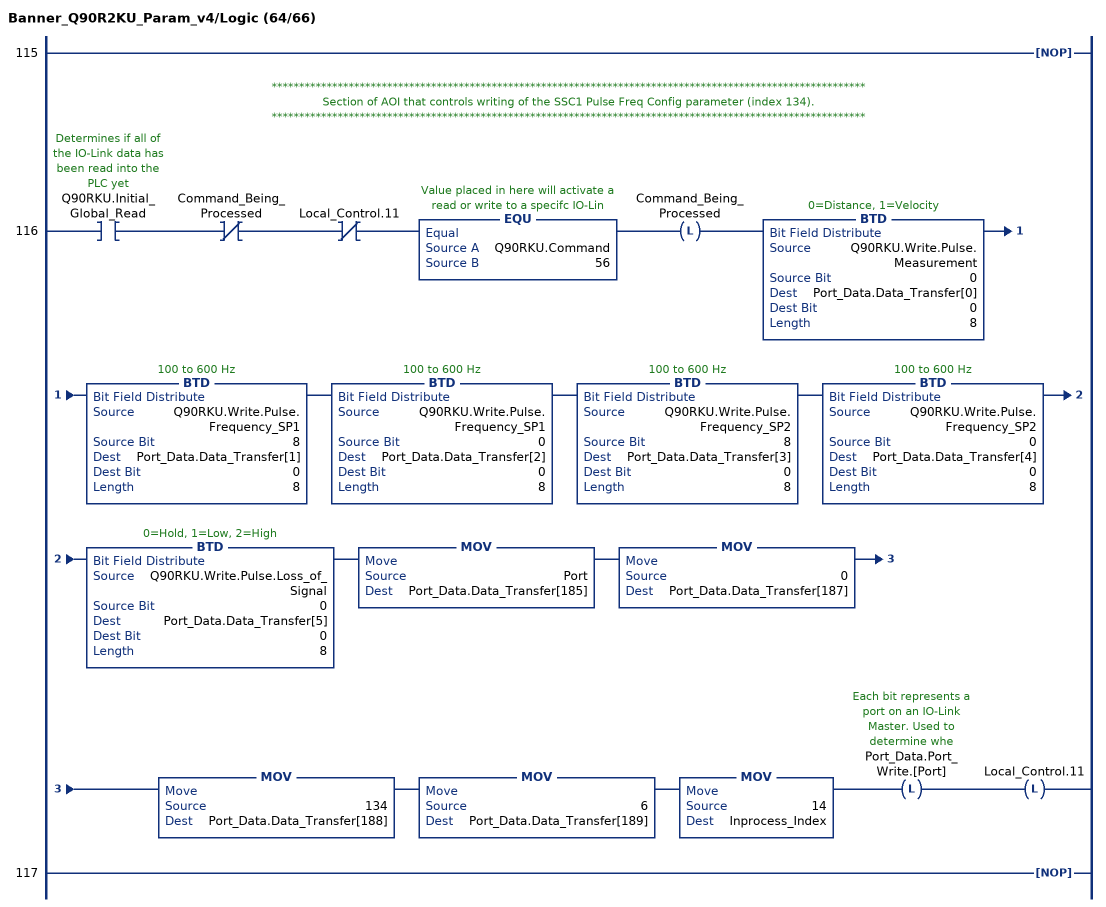
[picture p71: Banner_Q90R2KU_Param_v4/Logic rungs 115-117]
   115: NOP();
   // ************************************************************************************************************
   // Section of AOI that controls writing of the SSC1 Pulse Freq Config parameter (index 134).
   // ************************************************************************************************************
   116: XIC(Q90RKU.Initial_Global_Read)XIO(Command_Being_Processed)XIO(Local_Control.11)EQU(Q90RKU.Command,56)OTL(Command_Being_Processed)BTD(Q90RKU.Write.Pulse.Measurement,0,Port_Data.Data_Transfer[0],0,8)BTD(Q90RKU.Write.Pulse.Frequency_SP1,8,Port_Data.Data_Transfer[1],0,8)BTD(Q90RKU.Write.Pulse.Frequency_SP1,0,Port_Data.Data_Transfer[2],0,8)BTD(Q90RKU.Write.Pulse.Frequency_SP2,8,Port_Data.Data_Transfer[3],0,8)BTD(Q90RKU.Write.Pulse.Frequency_SP2,0,Port_Data.Data_Transfer[4],0,8)BTD(Q90RKU.Write.Pulse.Loss_of_Signal,0,Port_Data.Data_Transfer[5],0,8)MOV(Port,Port_Data.Data_Transfer[185])MOV(0,Port_Data.Data_Transfer[187])MOV(134,Port_Data.Data_Transfer[188])MOV(6,Port_Data.Data_Transfer[189])MOV(14,Inprocess_Index)OTL(Port_Data.Port_Write.[Port])OTL(Local_Control.11);
   117: NOP();
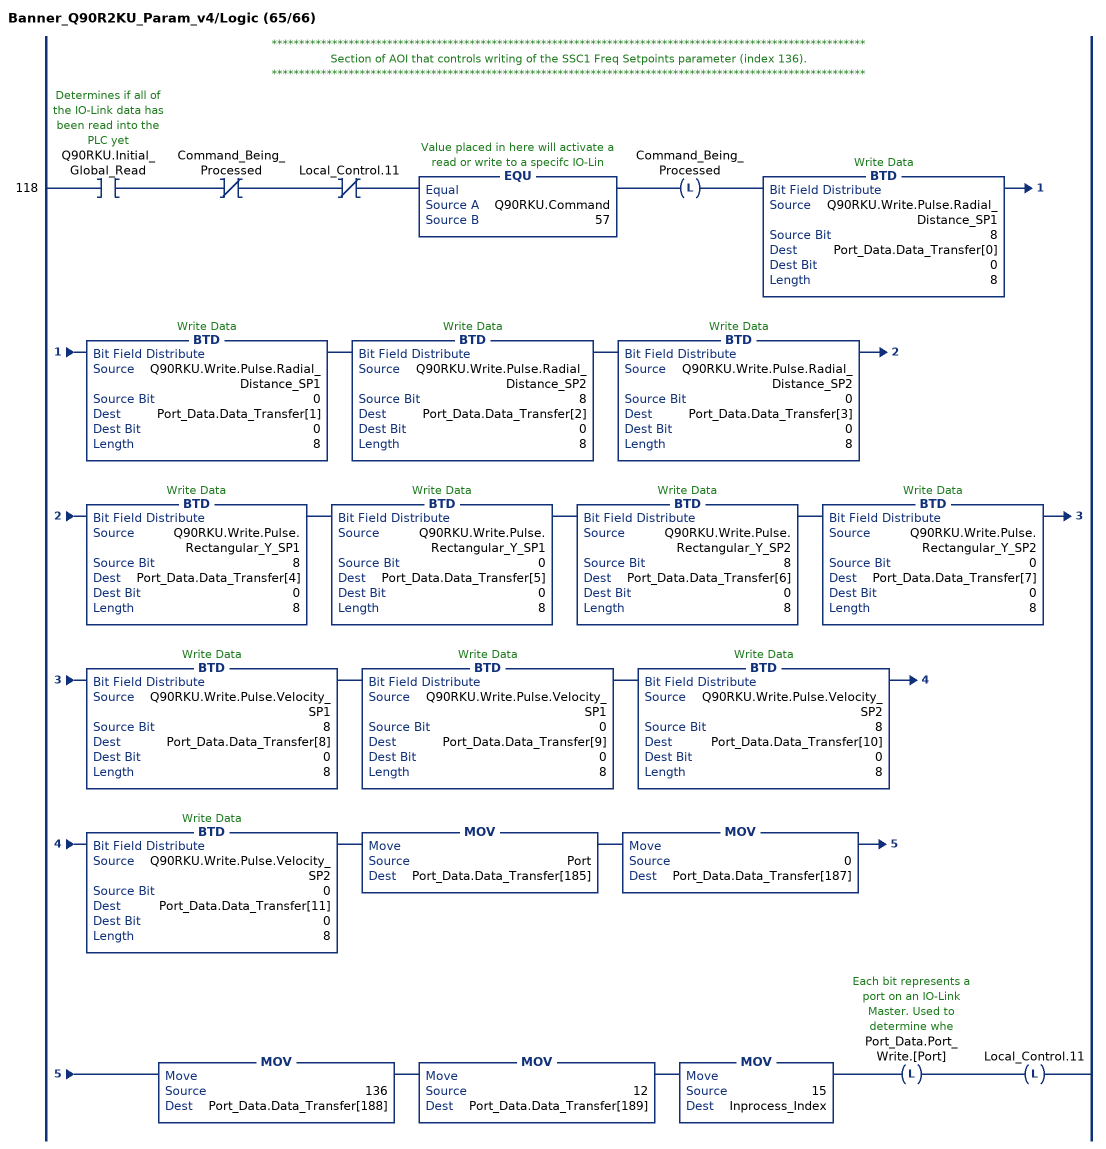
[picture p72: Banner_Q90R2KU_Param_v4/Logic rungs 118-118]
   // ************************************************************************************************************
   // Section of AOI that controls writing of the SSC1 Freq Setpoints parameter (index 136).
   // ************************************************************************************************************
   118: XIC(Q90RKU.Initial_Global_Read)XIO(Command_Being_Processed)XIO(Local_Control.11)EQU(Q90RKU.Command,57)OTL(Command_Being_Processed)BTD(Q90RKU.Write.Pulse.Radial_Distance_SP1,8,Port_Data.Data_Transfer[0],0,8)BTD(Q90RKU.Write.Pulse.Radial_Distance_SP1,0,Port_Data.Data_Transfer[1],0,8)BTD(Q90RKU.Write.Pulse.Radial_Distance_SP2,8,Port_Data.Data_Transfer[2],0,8)BTD(Q90RKU.Write.Pulse.Radial_Distance_SP2,0,Port_Data.Data_Transfer[3],0,8)BTD(Q90RKU.Write.Pulse.Rectangular_Y_SP1,8,Port_Data.Data_Transfer[4],0,8)BTD(Q90RKU.Write.Pulse.Rectangular_Y_SP1,0,Port_Data.Data_Transfer[5],0,8)BTD(Q90RKU.Write.Pulse.Rectangular_Y_SP2,8,Port_Data.Data_Transfer[6],0,8)BTD(Q90RKU.Write.Pulse.Rectangular_Y_SP2,0,Port_Data.Data_Transfer[7],0,8)BTD(Q90RKU.Write.Pulse.Velocity_SP1,8,Port_Data.Data_Transfer[8],0,8)BTD(Q90RKU.Write.Pulse.Velocity_SP1,0,Port_Data.Data_Transfer[9],0,8)BTD(Q90RKU.Write.Pulse.Velocity_SP2,8,Port_Data.Data_Transfer[10],0,8)BTD(Q90RKU.Write.Pulse.Velocity_SP2,0,Port_Data.Data_Transfer[11],0,8)MOV(Port,Port_Data.Data_Transfer[185])MOV(0,Port_Data.Data_Transfer[187])MOV(136,Port_Data.Data_Transfer[188])MOV(12,Port_Data.Data_Transfer[189])MOV(15,Inprocess_Index)OTL(Port_Data.Port_Write.[Port])OTL(Local_Control.11);
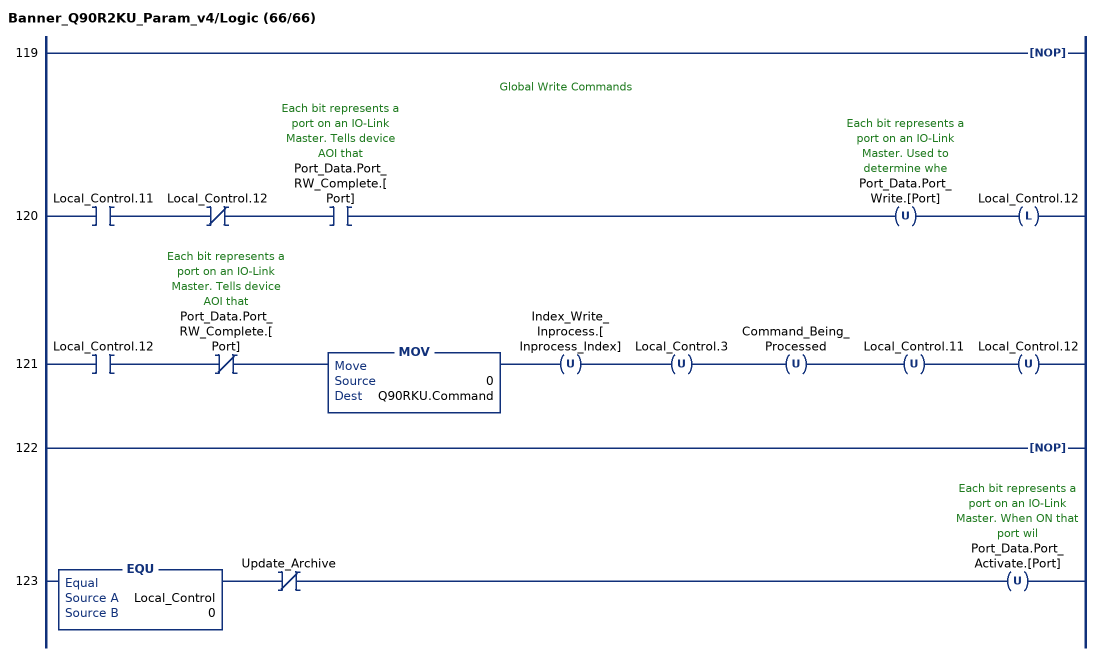
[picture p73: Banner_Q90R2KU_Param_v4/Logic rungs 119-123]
   119: NOP();
   // Global Write Commands
   120: XIC(Local_Control.11)XIO(Local_Control.12)XIC(Port_Data.Port_RW_Complete.[Port])OTU(Port_Data.Port_Write.[Port])OTL(Local_Control.12);
   121: XIC(Local_Control.12)XIO(Port_Data.Port_RW_Complete.[Port])MOV(0,Q90RKU.Command)OTU(Index_Write_Inprocess.[Inprocess_Index])OTU(Local_Control.3)OTU(Command_Being_Processed)OTU(Local_Control.11)OTU(Local_Control.12);
   122: NOP();
   123: EQU(Local_Control,0)XIO(Update_Archive)OTU(Port_Data.Port_Activate.[Port]);
END_ROUTINE
END_ADD_ON_INSTRUCTION
